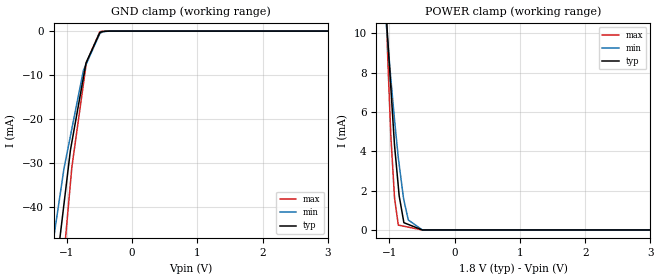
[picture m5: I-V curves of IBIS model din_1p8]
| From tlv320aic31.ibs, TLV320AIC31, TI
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|   din_1p8 Model
[Model]   din_1p8
Model_type   Input
Vinl = 0.54
Vinh = 1.26
|   typ   min   max
|   (nom PVT)   (fast PVT)   (slow PVT)
|C_comp from frequency sweep method (F=25MHz)
|Average
|C_comp   7.047e-12   6.870e-12   7.226e-12
|C_comp from LC tank measurement(L=1nH)
|Average
|Resonant Frequency(Hz)   2.070e+09   2.090e+09   2.060e+09
C_comp   5.917e-12   5.805e-12   5.975e-12
| Where nom  PVT is Nominal Process, 1.8V, 26C
|   Fast PVT is Strong Process,  1.98V, -40C
|   Slow PVT is Weak Process,   1.62V, 86C
[Model Spec]
|Subparameter   typ   min   max
Vinl   0.54   0.486   0.594
Vinh   1.26   1.134   1.386
[Voltage Range]   1.8   1.62   1.98
|Ambient Temperature   25   85   -40
|Junction Temperature
[Temperature Range]   26   86   -40
[Power Clamp Reference]   1.8   1.62   1.98
[GND Clamp Reference]   0   0   0
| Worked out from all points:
|   GND clamp passes 1 mA (typ) near -0.52 V on its own axis
|   POWER clamp passes 1 mA (typ) near -0.81 V on its own axis
[GND Clamp]
|   Voltage   I(typ)   I(min)   I(max)
-1.8V     -248.6mA   -142.9mA   -345.7mA
-1.215V   -60.5mA    -48.36mA   -81.14mA
-1.178V   -55.92mA   -44.66mA   -73.2mA
-1.043V   -39.19mA   -31.17mA   -50.81mA
-945mV    -27.02mA   -23.8mA    -34.49mA
-922.7mV  -25.17mA   -22.13mA   -30.84mA
-746.8mV  -10.54mA   -8.95mA    -12.06mA
-707.4mV  -7.264mA   -7.634mA   -7.852mA
-700.9mV  -7.053mA   -7.418mA   -7.16mA
-495mV    -338.9uA   -547.1uA   -147.5uA
-306.2mV  -2.612uA   -6.398uA   -288.4nA
3.6V      0A         0A         0A
[POWER Clamp]
|   Voltage   I(typ)   I(min)   I(max)
-1.8V     58.58mA    42.75mA    96.1mA
-1.073V   12.51mA    11.5mA     13.37mA
-1.033V   10.12mA    9.9mA      9.534mA
-1.022V   9.52mA     9.438mA    8.427mA
-976.1mV  7.154mA    7.627mA    4.701mA
-920.7mV  4.294mA    5.584mA    1.615mA
-863.3mV  2.217mA    3.671mA    247uA
-849.6mV  1.724mA    3.318mA    237.9uA
-777.6mV  369.1uA    1.512mA    189.6uA
-709.6mV  280.2uA    505.5uA    143.9uA
-494.1mV  18.66nA    1.306uA    0A
3.6V      0A         0A         0A
